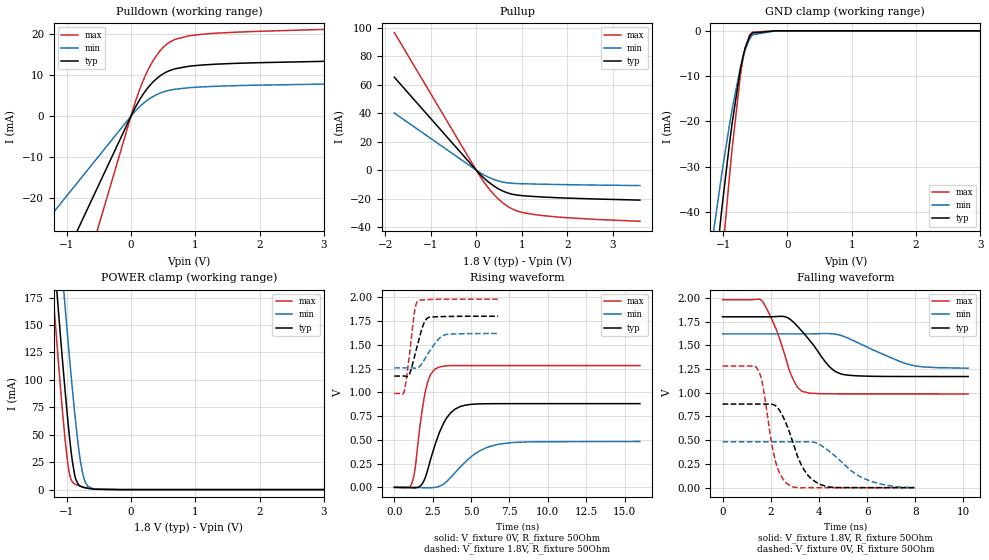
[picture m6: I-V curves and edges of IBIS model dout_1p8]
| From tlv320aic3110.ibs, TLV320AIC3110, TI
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|   dout_1p8 Model
[Model]   dout_1p8
Model_type   3-state
Polarity   Non-Inverting
Vmeas = 0.9
Vref = 0
Cref = 10pF
Rref = 100
|   typ   min   max
|   (nom PVT)   (fast PVT)   (slow PVT)
C_comp   1.531e-12   1.494e-12   1.585e-12
| Where nom  PVT is Nominal Process, 1.8V, 27C
|   Fast PVT is Strong Process,  1.98V, -40C
|   Slow PVT is Weak Process,   1.62V, 125C
[Voltage Range]   1.8   1.62   1.98
|Junction Temperature
[Temperature Range]   27   125   -40
[Pullup Reference]   1.8   1.62   1.98
[Pulldown Reference]   0   0   0
[Power Clamp Reference]   1.8   1.62   1.98
[GND Clamp Reference]   0   0   0
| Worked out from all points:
|   slope of the pulldown table from 0 to 0.27 V, typ, clamps not added: 38.1 ohm
|   slope of the pullup table from 0 to 0.27 V, typ, clamps not added: 32.3 ohm
|   GND clamp passes 1 mA (typ) near -0.58 V on its own axis
|   POWER clamp passes 1 mA (typ) near -0.65 V on its own axis
|   falling waveform, V_fixture 1.8V, R_fixture 50Ohm: 20-80 % time 1.16ns typ, 1.9ns min, 825ps max; typ from 1.8 V to 1.17 V
|   rising waveform, V_fixture 0V, R_fixture 50Ohm: 20-80 % time 1.15ns typ, 1.97ns min, 646ps max; typ from 0 V to 0.881 V
|   rising waveform, V_fixture 1.8V, R_fixture 50Ohm: 20-80 % time 619ps typ, 915ps min, 440ps max; typ from 1.17 V to 1.8 V
|   falling waveform, V_fixture 0V, R_fixture 50Ohm: 20-80 % time 825ps typ, 1.45ns min, 516ps max; typ from 0.881 V to 0 V
[Pulldown]
|   Voltage   I(typ)   I(min)   I(max)
-1.8V     -60.44mA   -35.18mA   -96.09mA
-85.32mV  -2.865mA   -1.668mA   -4.555mA
67.86mV   2.164mA    1.237mA    3.517mA
173.2mV   5mA        2.868mA    8.101mA
252.5mV   6.752mA    3.877mA    10.93mA
356.2mV   8.586mA    4.927mA    13.91mA
443.3mV   9.762mA    5.588mA    15.84mA
605.7mV   11.18mA    6.359mA    18.17mA
688.9mV   11.6mA     6.589mA    18.81mA
898.9mV   12.2mA     6.948mA    19.65mA
1.307V    12.71mA    7.299mA    20.29mA
3.598V    13.69mA    8.018mA    21.69mA
[GND Clamp]
|   Voltage   I(typ)   I(min)   I(max)
-1.8V     -229.5mA   -131.2mA   -348.8mA
-1.18V    -60.75mA   -47.37mA   -78.76mA
-1.019V   -39.14mA   -31.37mA   -50.91mA
-905.4mV  -25.36mA   -21.1mA    -32.68mA
-861.5mV  -20.53mA   -17.45mA   -26.18mA
-736.7mV  -8.878mA   -8.45mA    -10.44mA
-689.4mV  -5.55mA    -5.745mA   -6.036mA
-657.5mV  -3.753mA   -4.213mA   -3.76mA
-588.2mV  -1.219mA   -1.793mA   -923.6uA
-543.6mV  -475.1uA   -890.5uA   -286.4uA
-180mV    0A         -186nA     0A
3.598V    0A         0A         0A
[Pullup]
|   Voltage   I(typ)   I(min)   I(max)
-1.8V     65.35mA    40.15mA    96.77mA
67.14mV   -2.325mA   -1.411mA   -3.476mA
207.7mV   -6.661mA   -3.989mA   -10.05mA
360mV     -10.54mA   -6.205mA   -16.11mA
591.8mV   -14.82mA   -8.42mA    -23.2mA
720.7mV   -16.34mA   -9.058mA   -26.04mA
898.9mV   -17.53mA   -9.423mA   -28.71mA
1.331V    -18.66mA   -9.804mA   -31.46mA
1.981V    -19.63mA   -10.2mA    -33.43mA
3.598V    -21.07mA   -10.85mA   -35.98mA
[POWER Clamp]
|   Voltage   I(typ)   I(min)   I(max)
-1.8V     690.3mA    759.1mA    657.4mA
-1.215V   227.2mA    304.9mA    181.3mA
-1.183V   202.8mA    280.7mA    156.4mA
-1.137V   169.4mA    247.4mA    122.5mA
-1.032V   94.96mA    171.7mA    49.99mA
-959.4mV  49.54mA    122.1mA    15.25mA
-876.6mV  13.54mA    70.32mA    5.143mA
-816.7mV  4.428mA    38.71mA    3.695mA
-747mV    2.135mA    13.45mA    2.455mA
-674.1mV  1.217mA    3.078mA    1.394mA
-578.3mV  446.3uA    560.7uA    438.6uA
3.598V    0A         0A         0A
[Ramp]
R_load = 50
|   typ   min   max
dV/dt_r   0.528442/1.15095e-09   0.289603/1.96349e-09   0.768595/6.45673e-10
dV/dt_f   0.37756/1.159e-09   0.218018/1.90729e-09   0.595446/8.23787e-10
[Falling Waveform]
V_fixture = 1.8V
V_fixture_min = 1.62V
V_fixture_max = 1.98V
R_fixture = 50Ohm
|   Time   V(typ)   V(min)   V(max)
0s        1.8V       1.62V      1.98V
1.64ns    1.8V       1.62V      1.966V
2.231ns   1.803V     1.62V      1.665V
2.624ns   1.798V     1.62V      1.364V
2.992ns   1.731V     1.62V      1.11V
3.305ns   1.645V     1.62V      1.015V
4.456ns   1.27V      1.623V     988.5mV
4.941ns   1.196V     1.601V     988mV
7.834ns   1.171V     1.291V     987.6mV
10.2ns    1.171V     1.259V     987.6mV
[Rising Waveform]
V_fixture = 0V
V_fixture_min = 0V
V_fixture_max = 0V
R_fixture = 50Ohm
|   Time   V(typ)   V(min)   V(max)
0s        1.057nV    20.63nV    632.1pV
1.159ns   -4.763mV   68.5uV     50.16mV
1.351ns   -5.185mV   328.3uV    193.8mV
1.761ns   26.52mV    -2.734mV   755.5mV
2.056ns   121.3mV    -3.785mV   1.033V
2.369ns   297.9mV    -3.668mV   1.187V
2.848ns   538.7mV    6.729mV    1.26V
3.979ns   825.5mV    158.8mV    1.281V
6.812ns   880.4mV    454.1mV    1.281V
16ns      880.7mV    482.7mV    1.281V
[Rising Waveform]
V_fixture = 1.8V
V_fixture_min = 1.62V
V_fixture_max = 1.98V
R_fixture = 50Ohm
|   Time   V(typ)   V(min)   V(max)
0s        1.171V     1.257V     987.6mV
645ps     1.171V     1.257V     1.012V
951ps     1.18V      1.257V     1.352V
1.306ns   1.371V     1.254V     1.838V
1.55ns    1.522V     1.258V     1.965V
1.937ns   1.73V      1.338V     1.973V
2.251ns   1.789V     1.421V     1.976V
2.905ns   1.795V     1.564V     1.979V
3.351ns   1.797V     1.607V     1.98V
6.764ns   1.8V       1.619V     1.98V
[Falling Waveform]
V_fixture = 0V
V_fixture_min = 0V
V_fixture_max = 0V
R_fixture = 50Ohm
|   Time   V(typ)   V(min)   V(max)
0s        880.7mV    482.7mV    1.281V
1.472ns   880.7mV    482.7mV    1.242V
1.669ns   880.7mV    482.7mV    1.077V
1.987ns   881.2mV    482.7mV    542.8mV
2.202ns   862.7mV    482.7mV    274.1mV
2.693ns   641.8mV    482.7mV    39.18mV
3.276ns   237.1mV    482.6mV    -1.834mV
4.003ns   40.22mV    458.9mV    452.6uV
5.921ns   441.5uV    90.75mV    4uV
7.957ns   19.03uV    1.516mV    372.3nV
